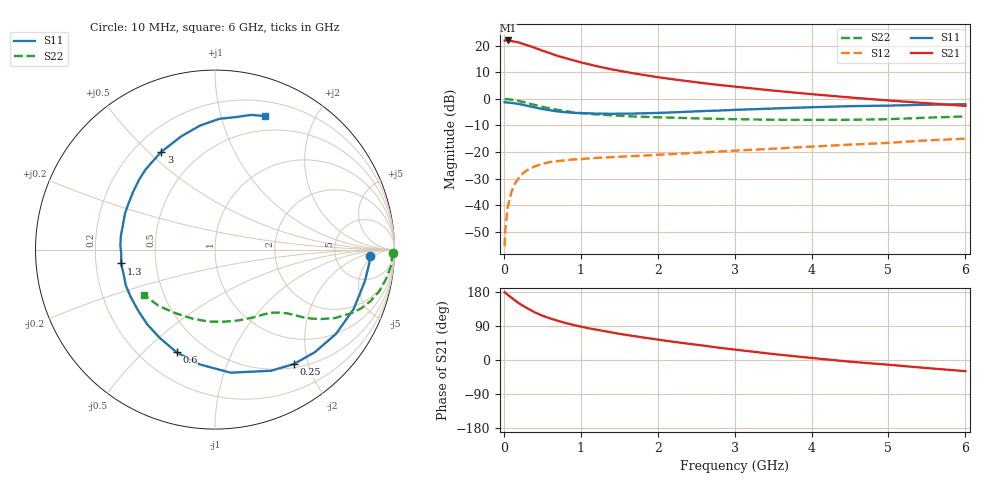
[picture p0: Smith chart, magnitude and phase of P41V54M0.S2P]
! SIEMENS Small Signal Semiconductors
! BFP182
! Si NPN RF Bipolar Junction Transistor in SOT143
! VCE = 1.5 V  IC = 4 mA
! Common Emitter S-Parameters:  March  1996
# GHz  S  MA  R  50
!  f  S11  S21  S12  S22
! GHz  MAG  ANG  MAG  ANG  MAG  ANG  MAG  ANG
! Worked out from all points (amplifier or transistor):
!   36 points, 10 MHz to 6 GHz, reference 50 ohm
!   highest |S21| = 22.0 dB at 50 MHz (marker M1)
!   |S21| within 3 dB of that: start of sweep to 424.6 MHz
!   unconditionally stable (mu >= 1): 1.667 GHz to 5.794 GHz
!   at 250 MHz: K = 0.19, MSG = 24.3 dB, |S12| = -27.9 dB
!   at 1.4 GHz: K = 0.89, MSG = 16.5 dB, |S12| = -21.9 dB
!   at 6 GHz: K = 0.98, MSG = 6.2 dB, |S12| = -15.0 dB
!   S11 on the Smith chart (normalised r, x): 10 MHz: 13, -4; 250 MHz: 0.55, -1.77; 600 MHz: 0.35, -0.64; 1.3 GHz: 0.31, -0.07; 3 GHz: 0.31, +0.55; 6 GHz: 0.34, +1.38
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0.01  0.8634 -2.4  12.45 178.7  0.0017 82.4  0.9915 -1.0
0.02  0.8633 -4.9  12.54 177.3  0.0036 90.8  0.9871 -1.9
0.05  0.8535 -11.9  12.56 172.0  0.0092 84.8  0.9863 -4.9
0.15  0.8216 -34.8  11.86 156.5  0.0264 70.8  0.9449 -14.1
0.2  0.7977 -45.8  11.46 149.2  0.0335 66.4  0.9129 -18.3
0.25  0.7742 -55.5  10.78 142.8  0.0402 60.9  0.8776 -21.9
0.3  0.7436 -65.2  10.27 137.2  0.0454 57.2  0.8411 -24.8
0.4  0.6912 -82.8  9.172 125.9  0.0536 49.6  0.7699 -29.7
0.5  0.645 -97.7  8.081 117.1  0.0601 43.8  0.7083 -33.1
0.6  0.6108 -110.5  7.231 109.9  0.065 39.8  0.6621 -35.5
0.7  0.5807 -121.9  6.427 103.6  0.0675 36.9  0.622 -37.4
0.8  0.5622 -132.2  5.858 97.7  0.0699 34.4  0.59 -38.8
0.9  0.5465 -141.6  5.342 92.8  0.0728 32.6  0.5624 -40.0
1.1  0.5358 -157.9  4.499 83.8  0.0759 30.3  0.5255 -42.3
1.3  0.5289 -171.6  3.855 76.4  0.0789 28.2  0.5008 -44.5
1.7  0.5302 166.2  3.004 62.9  0.0843 27.5  0.4661 -49.3
2.2  0.5577 145.1  2.337 48.2  0.0918 27.1  0.4435 -56.6
3  0.6215 118.8  1.705 27.5  0.1063 26.1  0.416 -71.6
3.5  0.6592 106.4  1.433 15.8  0.1157 24.9  0.405 -82.8
4.5  0.7293 88.0  1.064 -4.5  0.1379 21.5  0.4048 -108.3
5.5  0.7767 75.0  0.83 -21.3  0.1659 16.8  0.4432 -134.6
6  0.794 69.6  0.739 -29.5  0.1785 12.9  0.4684 -147.2
